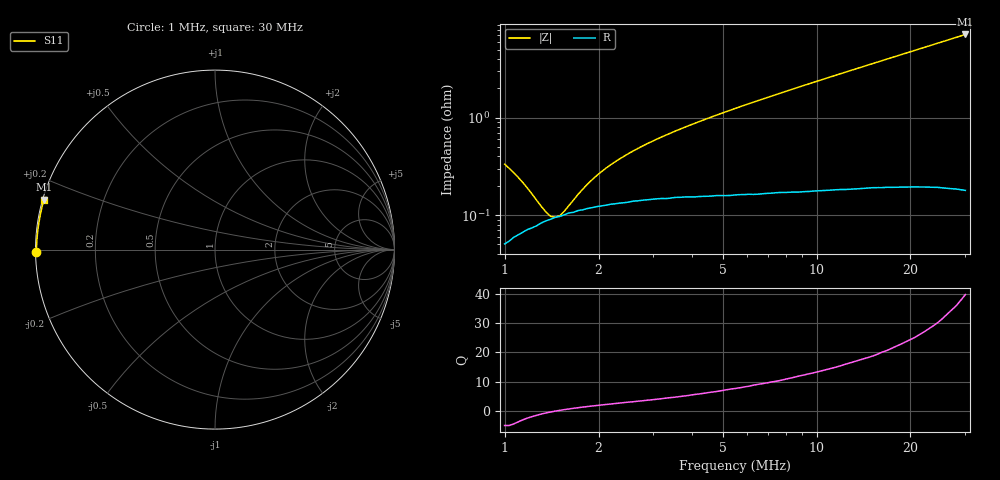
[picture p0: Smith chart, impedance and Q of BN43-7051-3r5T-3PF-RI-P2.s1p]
! ListType=Log
!!BN43-7051 3.5T 3PF Port 2
# MHz S RI R 50
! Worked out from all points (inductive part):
!   101 points, 1 MHz to 30 MHz, reference 50 ohm
!   read as one part to ground: L = 30.2 nH near 2.505 MHz
!   highest Q = 39.8 at 30 MHz (marker M1), where L = 37.8 nH
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1  -0.9979 -0.0131
1.070391  -0.9976 -0.0106
1.185376  -0.9971 -0.00694
1.312713  -0.9967 -0.00356
1.453729  -0.9962 -0.000316
1.556058  -0.996 0.00176
1.782833  -0.9955 0.00584
1.908328  -0.9952 0.00787
2.113327  -0.9949 0.011
2.505087  -0.9944 0.0163
3.072204  -0.9939 0.0232
3.767708  -0.9934 0.031
4.780527  -0.9928 0.0417
5.666721  -0.9922 0.0508
6.492571  -0.9917 0.059
8.52288  -0.99 0.0789
10.45234  -0.9881 0.0974
11.97563  -0.9864 0.1119
13.72092  -0.9843 0.1283
15.72057  -0.9815 0.1469
17.40932  -0.979 0.1626
19.27949  -0.9759 0.1799
21.35055  -0.9722 0.199
22.85344  -0.9693 0.2128
25.30843  -0.9643 0.2351
27.08991  -0.9603 0.2513
28.9968  -0.9559 0.2686
30  -0.9534 0.2777
